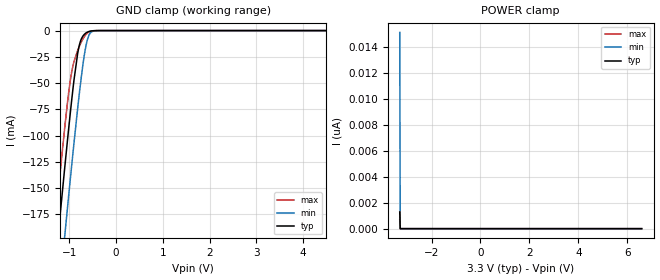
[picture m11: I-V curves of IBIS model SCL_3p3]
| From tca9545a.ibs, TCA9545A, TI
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|   Model
[Model]   SCL_3p3
Model_type   Input
Vinl = 0.99
Vinh = 2.31
|   typ   min   max
C_comp   3.453pF   3.557pF   3.722pF
[Voltage Range]   3.3   3   3.6
[Temperature Range]   27   125   -40
[Power Clamp Reference]   3.3   3   3.6
[GND Clamp Reference]   -0   -0   -0
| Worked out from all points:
|   GND clamp passes 1 mA (typ) near -0.59 V on its own axis
[GND Clamp]
|   Voltage   I(typ)   I(min)   I(max)
-3.3V     -1.2A      -1.262A    -1.16A
-1.379V   -259.7mA   -325.6mA   -218.8mA
-1.251V   -199.1mA   -264.8mA   -158.7mA
-1.231V   -189.8mA   -255.5mA   -149.6mA
-1.092V   -126.3mA   -191.3mA   -88.38mA
-953.7mV  -66.59mA   -128.9mA   -39.62mA
-825mV    -21.83mA   -74.21mA   -18.95mA
-765.6mV  -10.26mA   -51.1mA    -12.64mA
-696.3mV  -4.314mA   -27.51mA   -6.769mA
-607.2mV  -1.28mA    -7.279mA   -2.055mA
-409.2mV  -25.36uA   -76.43uA   -26.64uA
6.59V     0A         0A         0A
[POWER Clamp]
|   Voltage   I(typ)   I(min)   I(max)
-3.3V     1.289nA    15.15nA    694.8pA
-3.28V    0A         0A         0A
-3.27V    0A         0A         0A
6.59V     0A         0A         0A
